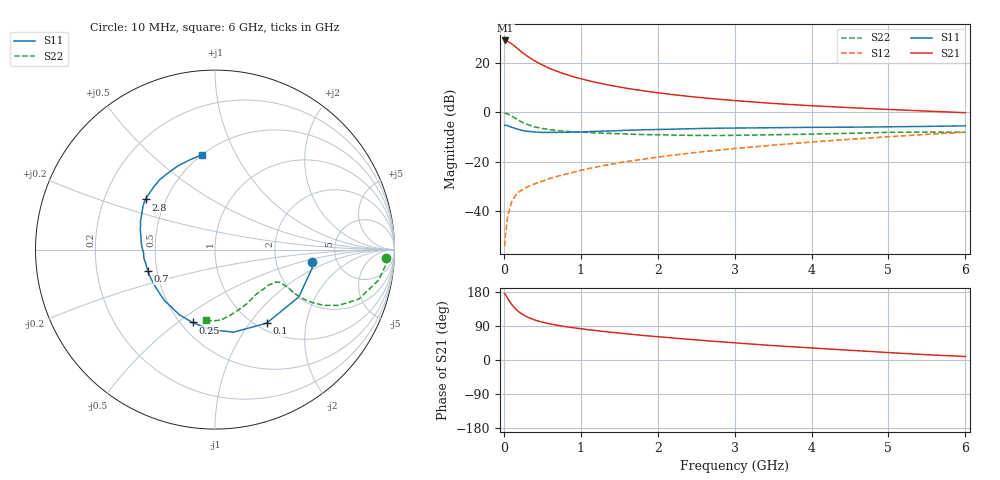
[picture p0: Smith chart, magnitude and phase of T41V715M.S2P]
! Infineon Technologies  Discrete & RF Semiconductors
! BFR182T
! Si NPN RF Bipolar Junction Transistor in SC75
! VCE = 1.75 V  IC = 15 mA
! Common Emitter S-Parameters:  October  1999
# GHz  S  MA  R  50
!  f  S11  S21  S12  S22
! GHz  MAG  ANG  MAG  ANG  MAG  ANG  MAG  ANG
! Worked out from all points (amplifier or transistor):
!   36 points, 10 MHz to 6 GHz, reference 50 ohm
!   highest |S21| = 29.3 dB at 20 MHz (marker M1)
!   |S21| within 3 dB of that: start of sweep to 166.4 MHz
!   unconditionally stable (mu >= 1): 658.7 MHz to 3.826 GHz
!   at 250 MHz: K = 0.61, MSG = 27.7 dB, |S12| = -31.3 dB
!   at 1.4 GHz: K = 1.14, MAG = 13.7 dB, |S12| = -21.1 dB
!   at 6 GHz: K = 0.86, MSG = 4.0 dB, |S12| = -8.0 dB
!   S11 on the Smith chart (normalised r, x): 10 MHz: 3.24, -0.63; 100 MHz: 1.11, -1.21; 250 MHz: 0.57, -0.57; 700 MHz: 0.44, -0.13; 2.8 GHz: 0.39, +0.28; 6 GHz: 0.50, +0.74
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0.01  0.543 -7.2  29.02 175.4  0.0019 77.6  0.9524 -2.8
0.02  0.5509 -10.8  29.09 172.9  0.0031 101.0  0.9613 -4.3
0.05  0.5364 -29.4  28 162.2  0.0077 83.4  0.9269 -10.6
0.1  0.5006 -54.9  24.95 147.3  0.015 71.1  0.847 -19.0
0.15  0.4718 -77.2  21.62 135.2  0.0204 64.9  0.7556 -24.3
0.2  0.4459 -93.8  18.65 126.3  0.0244 63.2  0.6804 -27.2
0.25  0.4248 -107.1  16.14 119.4  0.0271 59.6  0.618 -28.5
0.3  0.4141 -118.4  14.12 113.9  0.0303 59.9  0.5737 -29.1
0.4  0.3998 -135.2  11.22 105.7  0.0353 60.3  0.5074 -28.9
0.5  0.3916 -146.4  9.228 100.0  0.0398 61.8  0.4712 -27.9
0.6  0.3918 -155.5  7.8 95.3  0.0455 63.0  0.4454 -27.4
0.7  0.3931 -162.3  6.78 91.5  0.0503 64.4  0.4267 -27.0
0.9  0.3991 -173.4  5.342 85.3  0.0601 66.4  0.4022 -27.0
1.1  0.4066 178.4  4.423 79.8  0.072 67.7  0.3889 -27.9
1.3  0.4161 171.7  3.775 75.2  0.0832 68.7  0.3767 -29.4
1.6  0.4331 164.1  3.093 69.0  0.1002 69.4  0.3631 -32.2
2.2  0.456 153.0  2.298 58.0  0.1352 69.2  0.3467 -40.2
2.8  0.4774 144.2  1.849 48.3  0.171 67.5  0.3384 -49.5
3.5  0.4881 134.3  1.522 38.0  0.2156 65.0  0.3511 -60.7
4.5  0.5003 121.7  1.25 25.7  0.2839 59.8  0.3761 -77.3
5.5  0.5193 105.7  1.063 13.9  0.3576 53.2  0.3974 -91.5
6  0.5334 98.0  0.986 9.2  0.3965 49.2  0.3952 -97.6
